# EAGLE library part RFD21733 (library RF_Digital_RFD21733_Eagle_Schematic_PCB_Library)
RFD21733 RFDP8 Datasheet: http://www.rfdigital.com/wp-content/uploads/2014/03/RFDP8.RF_.Modules.Manual.pdf
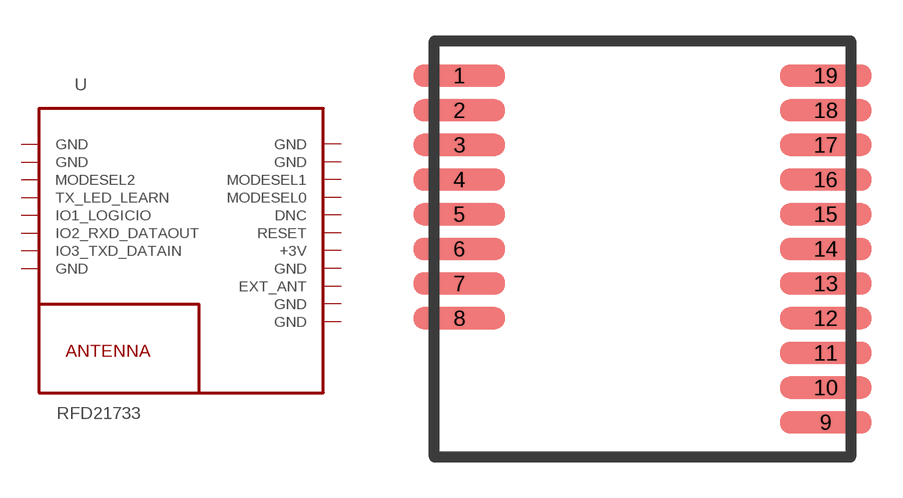
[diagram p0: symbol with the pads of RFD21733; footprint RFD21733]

Designator prefix U

## RFD21733  [RFD21733]
1  GND  pwr
2  GND  pwr
3  MODESEL2  in
4  TX_LED_LEARN
5  IO1_LOGICIO
6  IO2_RXD_DATAOUT
7  IO3_TXD_DATAIN
8  GND  pwr
9  GND  pwr
10  GND  pwr
11  EXT_ANT  nc
12  GND  pwr
13  +3V  pwr
14  RESET
15  DNC  nc
16  MODESEL0  in
17  MODESEL1  in
18  GND  pwr
19  GND  pwr

## Footprint RFD21733 (pad centres in mm)
RFD21733 PCB Layout
smd 3.353 x 0.813: 1 -6.706,7.62; 2 -6.706,6.35; 3 -6.706,5.08; 4 -6.706,3.81; 5 -6.706,2.54; 6 -6.706,1.27; 7 -6.706,0; 8 -6.706,-1.27; 9 6.706,-5.08; 10 6.706,-3.81; 11 6.706,-2.54; 12 6.706,-1.27; 13 6.706,0; 14 6.706,1.27; 15 6.706,2.54; 16 6.706,3.81; 17 6.706,5.08; 18 6.706,6.35; 19 6.706,7.62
